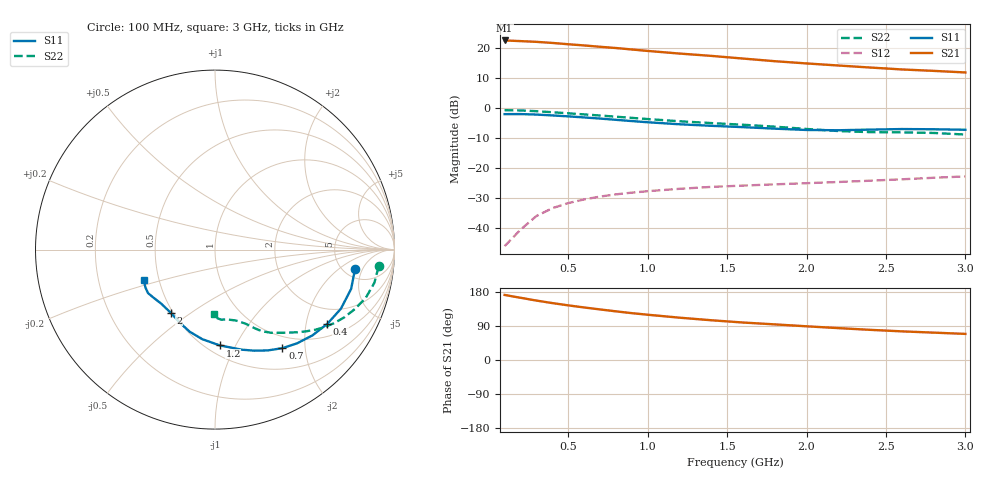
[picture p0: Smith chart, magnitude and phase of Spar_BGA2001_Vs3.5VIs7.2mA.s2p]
! Filename: 3_5G1.001
! Title: BGA2001 X0297-20 HFE=80
! Bias: Vce=3.5V,Ic=7.2mA
! Company: NXP Semiconductors NL
! User: Quality&Reliability T&D
! Measure time: 23 Oct 1998 / 09:20:53
#  MHz  S  MA  R 50
! Freq  S11  S21  S12  S22  :
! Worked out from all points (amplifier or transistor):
!   20 points, 100 MHz to 3 GHz, reference 50 ohm
!   highest |S21| = 22.4 dB at 100 MHz (marker M1)
!   |S21| within 3 dB of that: start of sweep to 900.7 MHz
!   unconditionally stable (mu >= 1): 1.929 GHz to end of sweep
!   at 400 MHz: K = 0.26, MSG = 27.5 dB, |S12| = -33.4 dB
!   at 1.2 GHz: K = 0.63, MSG = 22.5 dB, |S12| = -26.9 dB
!   at 3 GHz: K = 1.24, MAG = 14.3 dB, |S12| = -22.8 dB
!   S11 on the Smith chart (normalised r, x): 100 MHz: 6.33, -3.60; 400 MHz: 1.40, -2.65; 700 MHz: 0.81, -1.59; 1.2 GHz: 0.58, -0.87; 2 GHz: 0.49, -0.42; 3 GHz: 0.41, -0.17
100  0.7877 -7.9  13.23 171.7  0.005022 57.8  0.9166 -5.9
200  0.7895 -16.1  12.9 164.2  0.009435 78.6  0.9072 -11.7
300  0.775 -25.2  12.54 156.9  0.01592 78.0  0.8819 -17.8
400  0.75 -33.6  12.03 150.2  0.02148 73.5  0.847 -23.0
500  0.7234 -41.3  11.44 144.2  0.02612 69.3  0.8136 -27.6
600  0.6943 -48.8  10.93 138.7  0.03007 66.0  0.7797 -31.7
700  0.6652 -55.6  10.38 133.5  0.0335 63.1  0.7472 -35.4
800  0.6337 -62.5  9.904 128.4  0.03648 60.6  0.7146 -38.7
900  0.6041 -68.8  9.367 123.6  0.03898 58.7  0.6828 -41.8
1000  0.5774 -75.0  8.858 119.5  0.04122 57.1  0.6527 -44.9
1200  0.5345 -87.1  8.012 111.7  0.04513 54.7  0.5995 -50.6
1400  0.5039 -98.1  7.328 104.9  0.04858 53.2  0.5596 -55.9
1600  0.4785 -107.2  6.615 98.9  0.05108 52.9  0.5247 -60.1
1800  0.4518 -115.7  5.978 94.0  0.05357 53.8  0.4878 -63.5
2000  0.4296 -125.2  5.486 88.9  0.056 53.9  0.4465 -67.6
2200  0.4248 -134.9  5.07 84.1  0.05862 53.9  0.4124 -73.4
2400  0.4353 -142.2  4.692 79.6  0.06156 54.6  0.3952 -80.0
2600  0.4449 -147.0  4.359 75.6  0.06499 56.3  0.3919 -84.9
2800  0.4414 -151.4  4.127 72.2  0.06891 56.8  0.3832 -87.9
3000  0.4329 -156.7  3.884 68.9  0.07256 57.6  0.3603 -91.0
